TYPE VAT_IN :
STRUCT
	Actual_Pressure	:	REAL	;
	Pressure_Sensor_1	:	REAL	;
	Pressure_Sensor_2	:	REAL	;
	Actual_Position	:	REAL	;
	Control_Mode	:	SINT	;			(*
											CONTROL MODE:	
											1=HOMING
											2=POSITION
											3=CLOSE
											4=OPEN
											5=PRESSURE
											6=HOLD:KEEP IN CURRENT POSITION
											7=LEARN:INTERNAL LEARN PROCEDURE
											*)
	Error_Number	:	UINT	;
	General_Status	:	UINT	;			(*
											BIT 0	FIELDBUS DATA VALID 
													0 = Valve is not in the EtherCAT state OPERATIONAL or the process data output 
													watchdog 
													(SyncManager2) is disabled 
													1 = Valve is in the EtherCAT state OPERATIONAL and the process data output 
													watchdog 
													(SyncManager2) is enabled 
											BIT 1 ZERO ADJUST EXECUTED 
													ZERO ADJUST successful executed, active for 2 seconds 
											BIT 2 PING PONG RX-BIT 
													PING PONG RX BIT, is inverted and transmitted back to the fieldbus master (PLC) 
											BIT 3 PRESSURE SIMULATION 
													0 = off 
													1 = on 
											BIT 4 TARGET PRESSURE REACHED 
													0 = The actual pressure is not within 2% of the pressure setpoint 
													1 = The actual pressure is within 2% of the pressure setpoint 
											BIT 5-6 NOT USED (reserved) - 
											BIT 7-8 ACCESS MODE 
											bit 8	bit 7
												0 		0 	= LOCAL 
												0 		1 	= REMOTE 
												1 		0 	= LOCKED 
											BIT 9 WARNINGS ACTIVE 
													0 = No WARNINGS 
													1 = At least one WARNING of the warning bitmaps is active (GENERAL 
														WARNING bitmap and EXTENDED WARNING bitmap) 
											BIT 10 SEALING STATE 
													Only valid if a sealing functionality is available.
													0 = valve is not sealed 
													1 = valve is sealed 
											BIT 11 INTERLOCK ACTIVE 
													Is set if an interlock input is active 
											BIT 12-15 NOT USED (reserved) -
											*)
	General_Warnings	:	UINT	;		(*
											BIT 0 NOT USED (reserved) - 
											BIT 1 LEARN DATA SET 
													Learn data not present. Learn required for adaptive pressure control. 
													Just active if adaptive pressure control algorithm is choosen. 
											BIT 2 NOT USED (reserved) - 
											BIT 3 POWER FAILURE BATTERY 
													Not ready, voltage too low. 
													Just active if power failure is available. 
											4-15 NOT USED (reserved) -
											*)
	Extended_Warnings	:	UINT	;		(*
											BIT 0 REMOTE CONTROL NOT POSSIBLE 
													Remote control not possible, access mode local is active, change to acces mode 
													remote or access mode locked 
											BIT 1 ACTUAL CONTROL MODE SETPOINT NOT ALLOWED 
													Not possible to switch the actual control mode to CONTROL MODE SETPOINT 
													• Control mode is interlock or fatal error 
													• CONTROL MODE SETPOINT is 5 (pressure) or 7 (learn) and no sensor 
													  is selected (sensor mode configuration) 
											BIT 2 ZERO DISABLED 
													Using zero function not possible 
											BIT 3 PFO DEACTIVATED 
													Power Failure Option is deactivated 
											BIT 4 NOT USED (reserved) - 
											BIT 5 OUT OF RANGE: PRESSURE SETPOINT 
													Value of PRESSURE SETPOINT is out of range 
											BIT 6 OUT OF RANGE: POSITION SETPOINT 
													Value of POSITION SETPOINT is out of range 
											BIT 7-9 NOT USED (reserved) - 
											BIT 10 OUT OF RANGE: CONTROL MODE SETPOINT 
													Value of CONTROL MODE SETPOINT is out of range 
											BIT 11 OUT OF RANGE: GENERAL CONTROL SETPOINT 
													Value of GENERAL CONTROL SETPOINT is out of range 
											BIT 12-15 NOT USED (reserved) -
											*)
END_STRUCT
END_TYPE
